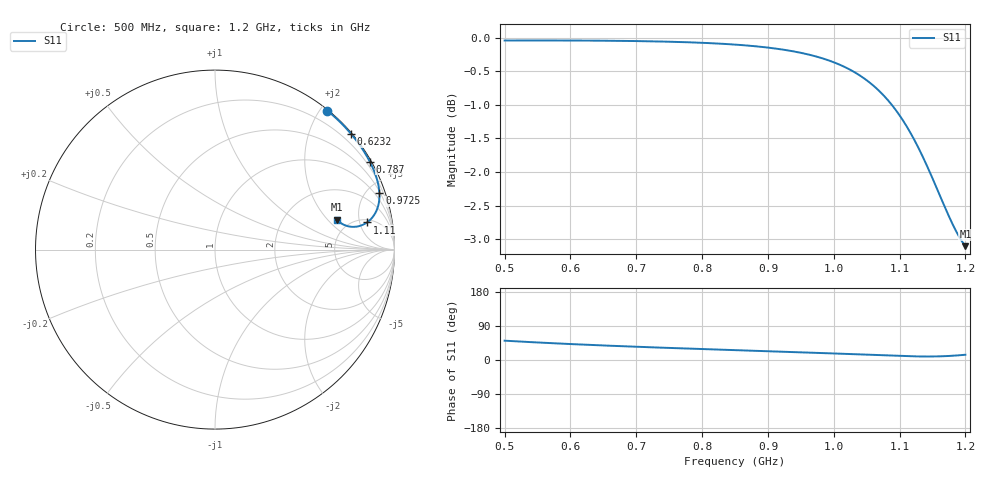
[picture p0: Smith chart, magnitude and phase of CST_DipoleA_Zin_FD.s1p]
! TOUCHSTONE file generated by CST MICROWAVE STUDIO
! Date and time: Fri Jan 17 08:39:40 2020
! Project name: Yang_RFID_1.cst
! Parameters = {d=9.936}
! Header version: 2015
! Port assignment regex: !\s*Touchstone port\s*([0-9]+)\s*=\s*CST MWS port\s*([0-9]+)\s*\(\"(.*)\"\)(\s*mode\s*([0-9]+))?.*
! Touchstone port assignment:
! Touchstone port 1 = CST MWS port 1 ("")
# GHz S MA R 50
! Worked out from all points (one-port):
!   1005 points, 500 MHz to 1.2 GHz, reference 50 ohm
!   lowest |S11| = -3.1 dB at 1.2 GHz (marker M1), VSWR 5.65, Z = 195 + j128 ohm
!   |S11| at or under -10 dB: nowhere
!   S11 on the Smith chart (normalised r, x): 500 MHz: 0.01, +2.10; 623.2 MHz: 0.02, +2.72; 787 MHz: 0.06, +3.78; 972.5 MHz: 0.58, +5.93; 1.11 GHz: 5.60, +6.55; 1.2 GHz: 3.90, +2.56
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0.5  0.9953 51.0
0.5455  0.9954 46.7
0.5875  0.9954 43.1
0.6232  0.9952 40.3
0.675  0.9947 36.6
0.7177  0.994 33.8
0.7625  0.9929 31.1
0.787  0.992 29.7
0.85  0.9884 26.1
0.8955  0.9839 23.5
0.9375  0.9772 21.1
0.9725  0.9686 19.0
0.9998  0.9589 17.2
1.0257  0.9462 15.6
1.0495  0.9301 13.9
1.0705  0.9114 12.5
1.0908  0.888 11.2
1.1097  0.8607 10.1
1.1125  0.8562 10.0
1.1251  0.8345 9.5
1.137  0.812 9.2
1.1475  0.791 9.2
1.158  0.7695 9.5
1.1678  0.7498 10.1
1.1776  0.7315 10.9
1.1916  0.7094 12.6
1.1965  0.7032 13.3
1.2  0.6994 13.8
